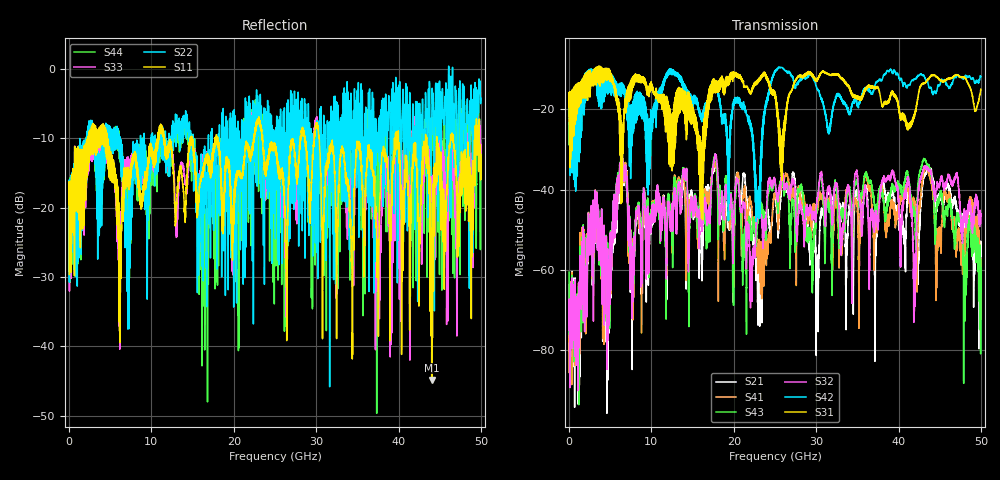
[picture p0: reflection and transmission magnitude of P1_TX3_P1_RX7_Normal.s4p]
!Keysight Technologies,N5225B,MY57041031,A.13.20.10
!Date: Friday, May 31, 2019 11:24:06
!Correction: S11(Full 4 Port(1,2,3,4))
!S12(Full 4 Port(1,2,3,4))
!S13(Full 4 Port(1,2,3,4))
!S14(Full 4 Port(1,2,3,4))
!S21(Full 4 Port(1,2,3,4))
!S22(Full 4 Port(1,2,3,4))
!S23(Full 4 Port(1,2,3,4))
!S24(Full 4 Port(1,2,3,4))
!S31(Full 4 Port(1,2,3,4))
!S32(Full 4 Port(1,2,3,4))
!S33(Full 4 Port(1,2,3,4))
!S34(Full 4 Port(1,2,3,4))
!S41(Full 4 Port(1,2,3,4))
!S42(Full 4 Port(1,2,3,4))
!S43(Full 4 Port(1,2,3,4))
!S44(Full 4 Port(1,2,3,4))
!S4P File: Measurements: <S11,S12,S13,S14>,
!<S21,S22,S23,S24>,
!<S31,S32,S33,S34>,
!<S41,S42,S43,S44>:
# Hz S  dB  R 50.0
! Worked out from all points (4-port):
!   5000 points, 10 MHz to 50 GHz, reference 50 ohm
!   strongest paths, dB at 10 MHz, 12.51 GHz, 25.01 GHz, 37.51 GHz, 50 GHz:
!     S31: -19.4, -27.0, -15.7, -14.5, -14.9
!     S42: -19.6, -10.0, -10.7, -12.9, -11.9
!     S32: -68.8, -43.5, -37.9, -48.1, -46.7
!     S43: -60.6, -44.0, -38.2, -42.0, -57.6
!     S41: -77.0, -44.2, -41.1, -46.4, -63.2
!     S21: -63.7, -43.6, -41.4, -44.1, -56.6
!   lowest |S11| = -44.8 dB at 44.03 GHz (marker M1), VSWR 1.01, Z = 49.7 + j0.506 ohm
!   |S11| at or under -10 dB: 4.66 GHz to 10.77 GHz (6.106 GHz wide, 79.2 % of centre); 23.49 GHz to 28.08 GHz (4.583 GHz wide, 17.8 % of centre); 30.37 GHz to 39.61 GHz (9.238 GHz wide, 26.4 % of centre)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
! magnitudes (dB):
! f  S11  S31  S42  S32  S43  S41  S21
! 10 MHz  -19.5  -19.4  -19.6  -68.8  -60.6  -77.0  -63.7
! 6.39 GHz  -20.9  -31.6  -14.4  -32.7  -32.6  -33.7  -34.1
! 21.25 GHz  -13.5  -14.3  -19.3  -43.4  -51.1  -39.7  -35.9
! 23.17 GHz  -7.6  -12.0  -38.2  -45.1  -43.3  -53.7  -65.9
! 25.51 GHz  -15.5  -23.7  -9.4  -39.5  -39.7  -43.0  -45.7
! 44.03 GHz  -44.8  -11.4  -15.3  -36.6  -37.4  -39.0  -35.7
! 50 GHz  -12.4  -14.9  -11.9  -46.7  -57.6  -63.2  -56.6
